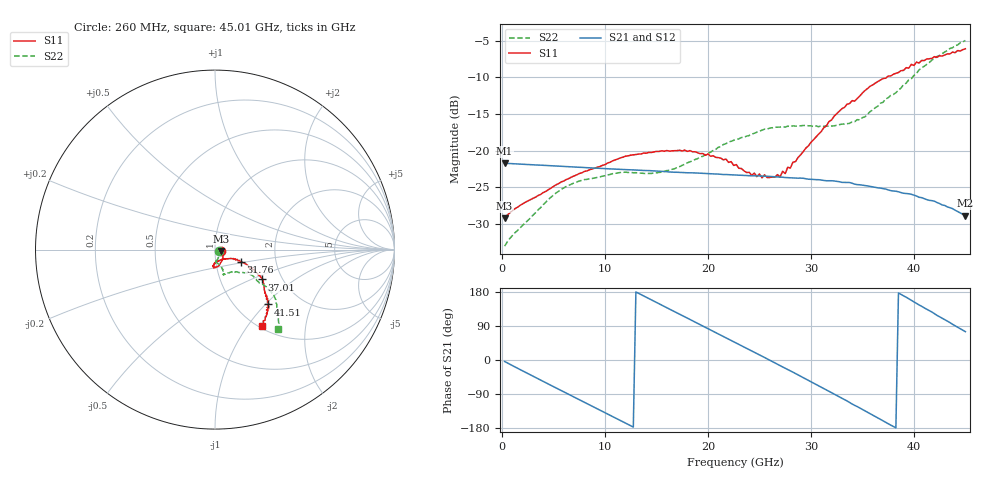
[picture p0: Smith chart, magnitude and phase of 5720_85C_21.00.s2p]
! Device:  ADRF5720
! Description: 0.5dB LSB GaAs MMIC 6-bit Digital Attenuator
! Frequency:  0.000009 -  40 GHz
! Ports:
!	RF1	= Port 1
!	RF2	= Port 2
! Vdd:  3.3 Volt
! Vss:  -3.3 Volt
! Control:  0/3.3 Volt
! State:  21.00 dB attenuation
! Data:  The device was measured using G-S-G Probes on a matrix board.
!  Data was collected using an calibrated 4 port network analyzer.
!  The reference plane for this measurement is at the launchers.
! Note:  Analog Devices supplies this data as a sample of measured data
!  for this product.  Your particular data for this product may vary.
!  Data was taken at 85 degrees C.
!  Analog Devices reserves the right to change this data at anytime.
# GHZ S DB R 45.0
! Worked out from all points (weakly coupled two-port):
!   180 points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, 260 MHz to 45.01 GHz, reference 45 ohm
!   highest |S21| = -21.73 dB at 260 MHz (marker M1); lowest = -28.9 dB at 45.01 GHz (marker M2)
!   lowest |S11| = -29.3 dB at 260 MHz (marker M3), VSWR 1.07, Z = 48.1 - j0.786 ohm
!   |S11| at or under -10 dB: start of sweep to 37.35 GHz
!   |S22| runs from -33.1 to -4.9 dB; largest |S21 - S12| = 0.00042
!   S11 on the Smith chart (normalised r, x): 260 MHz: 1.07, -0.02; 31.76 GHz: 1.32, -0.18; 37.01 GHz: 1.58, -0.58; 41.51 GHz: 1.39, -1.03; 45.01 GHz: 1.04, -1.16
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0.26  -29.25 -13.7  -21.73 -3.9  -21.72 -3.9  -33.06 -22.1
1.26  -27.94 -3.9  -21.81 -18.2  -21.80 -18.2  -31.23 -14.4
5.01  -24.89 -38.1  -22.08 -70.3  -22.07 -70.3  -26.07 -68.0
7.76  -23.04 -55.0  -22.29 -108.2  -22.28 -108.1  -24.07 -83.2
12.01  -20.76 -75.6  -22.60 -166.6  -22.58 -166.5  -22.95 -92.4
15.26  -20.12 -87.5  -22.81 148.3  -22.79 148.4  -22.98 -86.3
18.26  -20.00 -94.5  -23.03 107.0  -23.02 107.2  -21.53 -75.7
22.76  -21.91 -91.7  -23.34 44.7  -23.32 44.9  -18.49 -69.2
24.26  -23.38 -84.9  -23.45 24.0  -23.43 24.2  -17.76 -69.8
27.01  -23.61 -53.9  -23.60 -14.7  -23.58 -14.4  -16.79 -70.5
27.26  -22.82 -48.9  -23.64 -18.3  -23.63 -18.0  -16.75 -71.2
27.51  -23.14 -47.5  -23.68 -21.7  -23.67 -21.4  -16.78 -70.6
27.76  -22.27 -42.7  -23.70 -25.2  -23.68 -24.9  -16.66 -71.4
28.01  -22.39 -42.6  -23.73 -28.8  -23.71 -28.5  -16.71 -71.0
30.26  -18.52 -27.5  -23.94 -60.6  -23.92 -60.4  -16.74 -69.6
31.76  -16.04 -25.3  -24.12 -82.1  -24.10 -81.8  -16.68 -65.3
34.76  -12.53 -27.8  -24.67 -126.8  -24.65 -126.5  -15.80 -49.2
37.01  -10.16 -32.4  -25.20 -160.5  -25.18 -160.2  -13.40 -36.7
37.76  -9.81 -34.0  -25.47 -171.9  -25.45 -171.4  -12.47 -35.4
41.51  -7.45 -46.1  -26.80 130.2  -26.78 130.7  -7.96 -37.1
43.51  -6.79 -50.4  -27.80 98.7  -27.78 99.1  -6.05 -45.0
45.01  -6.09 -58.5  -28.89 74.8  -28.87 75.2  -4.95 -51.9
